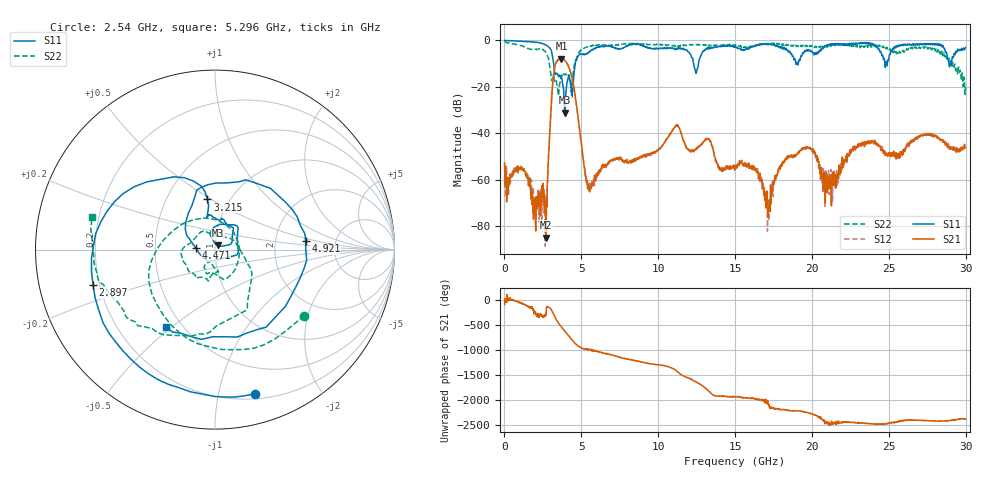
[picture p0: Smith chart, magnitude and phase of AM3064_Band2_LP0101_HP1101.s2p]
# Hz S DB R 50.0
!freq dBS11 angS11 dBS21 angS21 dBS12 angS12 dBS22 angS22
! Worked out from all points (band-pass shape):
!   1600 points, 10 MHz to 29.98 GHz, reference 50 ohm
!   highest |S21| = -7.82 dB at 3.703 GHz (marker M1); lowest = -84.8 dB at 2.69 GHz (marker M2)
!   |S21| within 3 dB of the highest: 3.292 GHz to 4.139 GHz (846.9 MHz wide, 22.8 % of centre)
!   lowest |S11| = -31.1 dB at 3.927 GHz (marker M3), VSWR 1.06, Z = 51.5 + j2.38 ohm
!   |S11| at or under -10 dB: 3.201 GHz to 4.602 GHz (1.401 GHz wide, 35.9 % of centre); 12.3 GHz to 12.62 GHz (322.8 MHz wide, 2.59 % of centre); 28.91 GHz to 29.08 GHz (166.1 MHz wide, 0.573 % of centre)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
!   |S22| runs from -23.7 to -0.2 dB; largest |S21 - S12| = 0.011
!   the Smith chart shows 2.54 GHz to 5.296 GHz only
!   S11 on the Smith chart (normalised r, x): 2.54 GHz: 0.24, -1.29; 2.897 GHz: 0.17, -0.14; 3.215 GHz: 0.79, +0.48; 4.471 GHz: 0.81, +0.01; 4.921 GHz: 3.00, +0.37; 5.296 GHz: 0.41, -0.48
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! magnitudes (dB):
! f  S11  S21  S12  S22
! 10 MHz  0.0  -52.8  -52.6  -0.2
! 2.54 GHz  -1.6  -67.2  -62.4  -4.2
! 2.69 GHz  -2.0  -84.8  -75.7  -5.1
! 2.897 GHz  -3.0  -45.7  -45.9  -8.9
! 3.215 GHz  -11.0  -13.5  -13.7  -15.8
! 3.703 GHz  -16.0  -7.8  -7.9  -15.5
! 3.927 GHz  -31.1  -8.6  -8.6  -14.8
! 4.471 GHz  -19.4  -18.8  -18.6  -14.1
! 4.921 GHz  -5.9  -40.1  -40.0  -4.4
! 5.015 GHz  -6.1  -45.0  -45.1  -4.2
! 5.296 GHz  -5.8  -59.7  -59.8  -3.0
! 10 GHz  -3.5  -47.2  -47.1  -1.9
! 11.24 GHz  -3.7  -36.7  -36.4  -2.6
! 15 GHz  -2.6  -54.6  -55.0  -2.0
! 16.37 GHz  -2.0  -55.5  -55.9  -2.3
! 17.14 GHz  -1.6  -73.0  -72.3  -1.4
! 18.25 GHz  -3.9  -51.9  -51.5  -1.9
! 19.99 GHz  -4.7  -46.7  -47.2  -2.2
! 21.13 GHz  -1.6  -57.8  -57.2  -2.6
! 23.18 GHz  -1.0  -45.1  -44.6  -2.8
! 25 GHz  -8.2  -48.7  -48.6  -3.2
! 29.98 GHz  -3.1  -46.1  -46.4  -20.3
